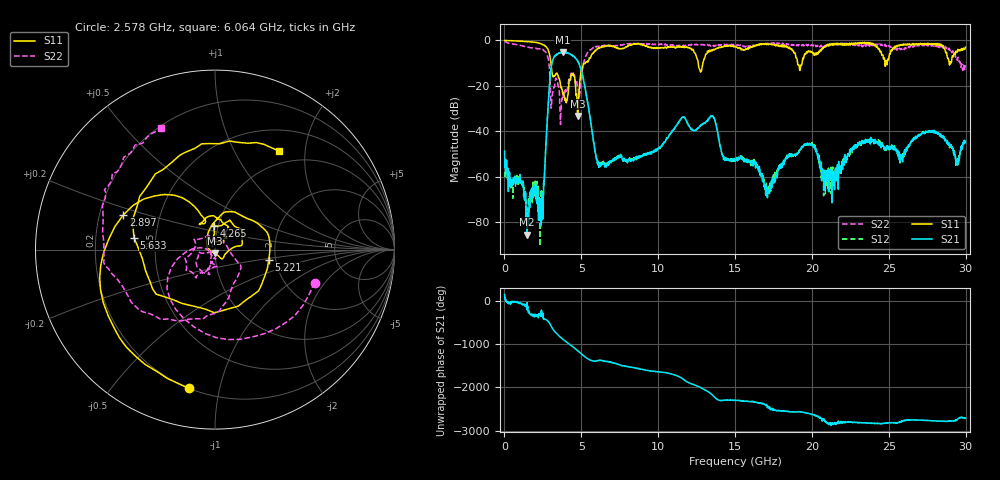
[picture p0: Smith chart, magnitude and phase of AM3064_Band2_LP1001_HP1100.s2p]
# Hz S DB R 50.0
!freq dBS11 angS11 dBS21 angS21 dBS12 angS12 dBS22 angS22
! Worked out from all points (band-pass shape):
!   1600 points, 10 MHz to 29.98 GHz, reference 50 ohm
!   highest |S21| = -5.19 dB at 3.777 GHz (marker M1); lowest = -85.6 dB at 1.472 GHz (marker M2)
!   |S21| within 3 dB of the highest: 3.173 GHz to 4.669 GHz (1.496 GHz wide, 38.2 % of centre)
!   lowest |S11| = -33.3 dB at 4.752 GHz (marker M3), VSWR 1.04, Z = 49.9 - j2.15 ohm
!   |S11| at or under -10 dB: 3.021 GHz to 5.262 GHz (2.241 GHz wide, 54.1 % of centre); 12.6 GHz to 12.91 GHz (305.3 MHz wide, 2.39 % of centre); 19.07 GHz to 19.36 GHz (290.6 MHz wide, 1.51 % of centre)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
!   |S22| runs from -37.1 to -0.3 dB; largest |S21 - S12| = 0.016
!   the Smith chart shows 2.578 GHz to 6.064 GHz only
!   S11 on the Smith chart (normalised r, x): 2.578 GHz: 0.20, -0.81; 2.897 GHz: 0.30, +0.17; 4.265 GHz: 0.96, +0.26; 5.221 GHz: 1.84, -0.23; 5.633 GHz: 0.38, +0.06; 6.064 GHz: 0.80, +1.54
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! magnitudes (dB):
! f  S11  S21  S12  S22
! 10 MHz  -0.1  -48.9  -60.3  -0.3
! 1.472 GHz  -0.6  -85.6  -78.8  -3.0
! 1.922 GHz  -0.8  -63.5  -62.7  -3.5
! 2.353 GHz  -1.5  -73.2  -67.3  -3.9
! 2.578 GHz  -2.1  -62.0  -62.7  -4.7
! 2.897 GHz  -5.3  -22.7  -22.7  -10.3
! 3.178 GHz  -16.1  -8.1  -8.1  -21.8
! 3.777 GHz  -23.0  -5.2  -5.4  -26.2
! 4.265 GHz  -17.6  -6.0  -6.0  -16.8
! 4.752 GHz  -33.3  -9.1  -9.0  -21.0
! 5.015 GHz  -12.9  -13.8  -13.8  -15.0
! 5.221 GHz  -10.3  -20.0  -20.0  -8.1
! 5.633 GHz  -6.8  -36.9  -37.0  -4.1
! 6.064 GHz  -3.7  -53.9  -53.7  -2.6
! 10 GHz  -3.4  -47.8  -47.4  -1.8
! 13.49 GHz  -4.2  -33.5  -33.3  -2.3
! 15 GHz  -2.6  -53.3  -52.9  -1.8
! 17.14 GHz  -1.7  -66.3  -65.8  -1.3
! 19.99 GHz  -5.0  -46.2  -46.3  -1.9
! 20.91 GHz  -2.2  -58.6  -57.3  -2.5
! 25 GHz  -8.0  -47.2  -47.1  -2.3
! 29.98 GHz  -3.0  -44.4  -44.7  -10.9
